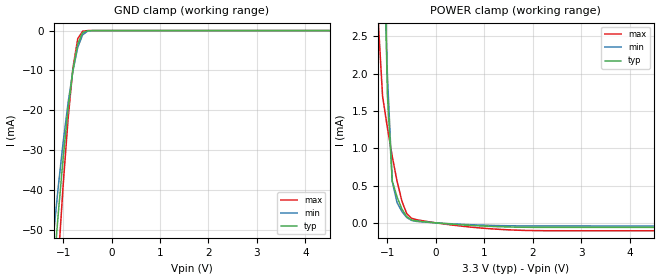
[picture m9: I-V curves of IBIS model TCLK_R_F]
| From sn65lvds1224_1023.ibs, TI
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|   Model TCLK_R_F
| Developed by Ayah Elkhordagy
[Model]   TCLK_R_F
Model_type   Input
Polarity   Non-Inverting
| Vinl and vih from datasheet
Vinl = 0.8
Vinh = 2.0
| C_comp values are extracted by ICX.
C_comp   0.86pF   0.833pF   0.86pF
[Temperature Range]   27   85   -40
[Voltage Range]   3.3V   3.0V   3.6V
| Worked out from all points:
|   GND clamp passes 1 mA (typ) near -0.62 V on its own axis
|   POWER clamp passes 1 mA (typ) near -0.94 V on its own axis
[GND_clamp]
| voltage   I(typ)   I(min)   I(max)
-3.3V     -471.9mA   -392.6mA   -586.6mA
-1.2V     -60.85mA   -51.2mA    -77.79mA
-1.1V     -45.66mA   -38.99mA   -57.36mA
-1V       -31.84mA   -27.92mA   -38.62mA
-900mV    -19.77mA   -18.2mA    -22.25mA
-800mV    -9.979mA   -10.12mA   -9.43mA
-700mV    -3.364mA   -4.221mA   -2.063mA
-600mV    -566.5uA   -1.082mA   -162uA
-500mV    -49.21uA   -158.2uA   -5.2uA
-400mV    -2.74uA    -16.22uA   -100nA
6.6V      0A         0A         0A
[POWER_clamp]
| voltage   I(typ)   I(min)   I(max)
-3.3V     119.9mA    83.71mA    140.6mA
-1.2V     8.657mA    6.74mA     2.831mA
-1.1V     4.886mA    4.19mA     1.701mA
-1V       1.716mA    1.986mA    1.274mA
-900mV    560.9uA    555.1uA    891.1uA
-800mV    344.8uA    270.2uA    556.8uA
-700mV    183.6uA    151.2uA    290.1uA
-600mV    81.12uA    71.45uA    122.3uA
-500mV    38.41uA    32.36uA    61.05uA
500mV     -25.32uA   -18.54uA   -41.77uA
1.7V      -58.13uA   -40.53uA   -98.98uA
6.6V      -60.99uA   -42.84uA   -106.3uA
